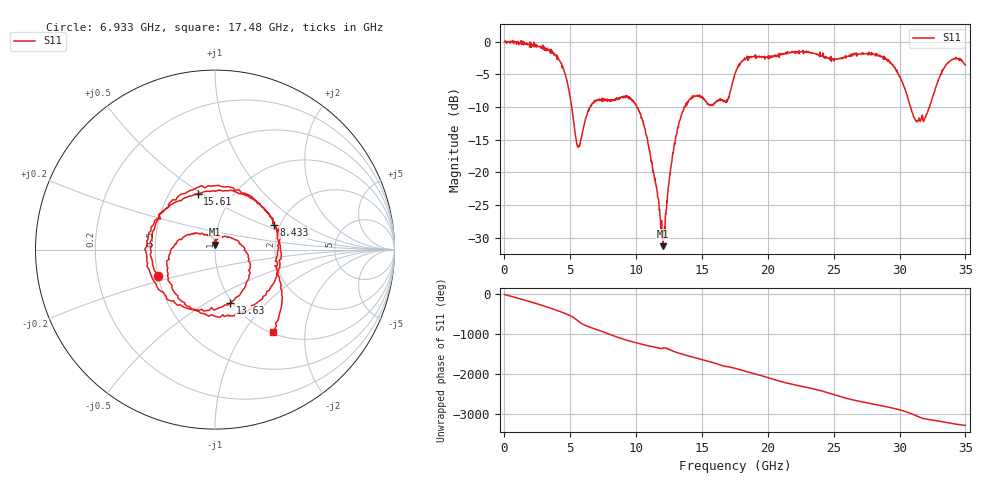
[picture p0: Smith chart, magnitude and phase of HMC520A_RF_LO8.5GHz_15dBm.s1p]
! Analog Devices, Inc.
! 1 Analog Way
! Wilmington, MA 01887
! http://www.analog.com
! Date:  2021-09-07 NN
! Board Name:  EV1HMC520ALC4 Revision A with HMC520ALC4 installed
! File Description:  S-Parameters for evaluation board without connectors or board loss de-embedded
! File Generation:  Calibrated Network Analyzer
! Chip Part Number:  HMC520A
! Chip Description:  GaAs, MMIC, IQ Mixer
! Chip Frequency:  6 to 10 GHz
! Chip Package:  LCC, 3.9 x 3.9 x 0.9 mm
! Chip State:
!  Temperature:  25C
!  LO Frequency:  8.5GHz
!  LO Power:  15dBm
! Note:
!  Analog Devices supplies this data as a sample of measured data at the evaluation board
!  ports for this product.  Your particular data for this product may vary.
!  Analog Devices reserves the right to change this data at anytime.
!  All lines below in this file are as is from the Network Analyzer.
!Keysight Technologies,N5245A,MY49151104,A.10.65.16
!Date: Wednesday, August 04, 2021 10:52:21
!Correction: S11(Full 2 Port(1,2))
!S1P File: Measurement: S11:
# Hz S  dB  R 50
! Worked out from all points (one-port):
!   1401 points, 10 MHz to 35 GHz, reference 50 ohm
!   lowest |S11| = -31.3 dB at 12.03 GHz (marker M1), VSWR 1.06, Z = 49.8 + j2.72 ohm
!   |S11| at or under -10 dB: 5.105 GHz to 6.512 GHz (1.408 GHz wide, 24.2 % of centre); 10.04 GHz to 13.65 GHz (3.609 GHz wide, 30.5 % of centre); 30.83 GHz to 32.28 GHz (1.454 GHz wide, 4.61 % of centre)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
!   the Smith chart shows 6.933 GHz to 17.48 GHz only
!   S11 on the Smith chart (normalised r, x): 6.933 GHz: 0.50, -0.16; 8.433 GHz: 1.87, +0.58; 13.63 GHz: 0.97, -0.64; 15.61 GHz: 0.69, +0.48; 17.48 GHz: 1.03, -1.37
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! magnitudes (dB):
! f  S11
! 10 MHz  0.0
! 3.084 GHz  -1.4
! 4.384 GHz  -4.0
! 4.834 GHz  -6.8
! 5.584 GHz  -16.2
! 6.933 GHz  -9.1
! 8.433 GHz  -8.9
! 8.758 GHz  -8.5
! 9.733 GHz  -9.0
! 10.48 GHz  -12.1
! 11.43 GHz  -20.9
! 12.03 GHz  -31.3
! 13.13 GHz  -13.4
! 13.63 GHz  -10.2
! 14.56 GHz  -8.3
! 15.61 GHz  -9.8
! 16.88 GHz  -8.9
! 17.48 GHz  -5.0
! 17.51 GHz  -5.0
! 18.41 GHz  -2.5
! 21.88 GHz  -1.6
! 26.25 GHz  -2.2
! 29 GHz  -2.7
! 30.63 GHz  -8.6
! 31.18 GHz  -11.9
! 31.73 GHz  -11.3
! 33.53 GHz  -3.6
! 35 GHz  -3.6
